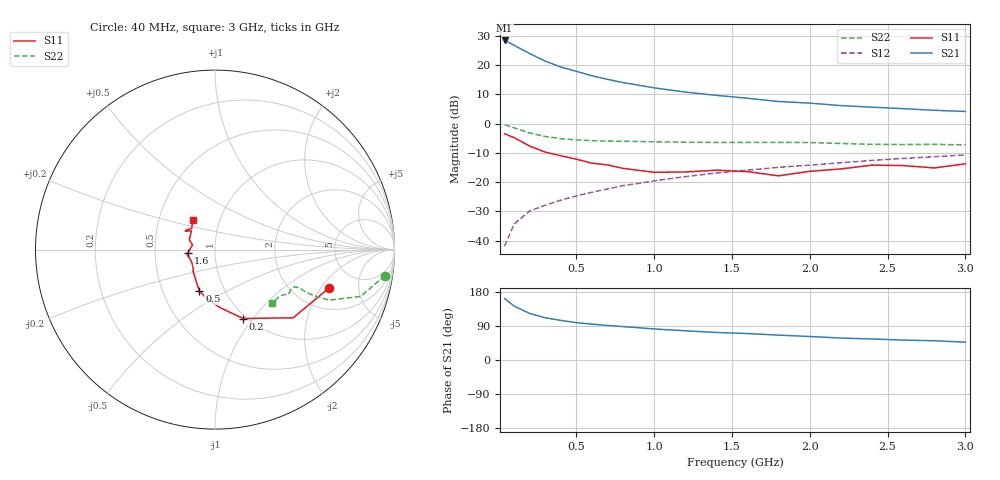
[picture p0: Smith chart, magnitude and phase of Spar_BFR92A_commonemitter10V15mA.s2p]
! Filename:  BFR92AI.S2P  Version:  2.0
! NXP part #: BFR92A  Date: May 1990
! Bias condition: Vce=10V, Ic=15mA
#  MHz  S  MA  R  50
! Freq  S11  S21  S12  S22  !GUM [dB]
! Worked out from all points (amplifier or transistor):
!   21 points, 40 MHz to 3 GHz, reference 50 ohm
!   highest |S21| = 28.5 dB at 40 MHz (marker M1)
!   |S21| within 3 dB of that: start of sweep to 148.3 MHz
!   unconditionally stable (mu >= 1): 897.4 MHz to 2.424 GHz; 2.693 GHz to 2.853 GHz
!   at 300 MHz: K = 0.77, MSG = 24.7 dB, |S12| = -28.0 dB
!   at 1 GHz: K = 1.01, MAG = 15.2 dB, |S12| = -19.6 dB
!   at 3 GHz: K = 0.98, MSG = 7.4 dB, |S12| = -10.7 dB
!   S11 on the Smith chart (normalised r, x): 40 MHz: 3.11, -2.41; 200 MHz: 0.97, -0.90; 500 MHz: 0.76, -0.37; 1.6 GHz: 0.74, -0.03; 3 GHz: 0.74, +0.25
40  0.672 -18.4  26.59 162.4  0.008 77.9  0.958 -8.7
100  0.578 -41.1  22.06 142.4  0.019 69.8  0.853 -17.8
200  0.415 -67.7  15.88 123.0  0.032 69.8  0.695 -23.9
300  0.326 -84.7  11.83 111.6  0.04 68.6  0.604 -25.0
400  0.283 -97.6  9.353 104.5  0.049 70.2  0.555 -25.1
500  0.247 -110.7  7.884 98.6  0.058 70.0  0.527 -24.5
600  0.211 -119.1  6.622 94.7  0.067 71.7  0.512 -24.5
700  0.197 -123.3  5.747 91.3  0.076 73.6  0.503 -24.7
800  0.172 -135.1  5.06 88.1  0.087 73.4  0.499 -24.6
900  0.159 -139.5  4.561 85.2  0.095 74.8  0.496 -25.0
1000  0.147 -152.9  4.106 82.0  0.105 74.6  0.489 -25.1
1200  0.149 -160.4  3.476 77.1  0.124 74.6  0.482 -26.1
1400  0.16 -172.5  3.055 72.7  0.143 74.2  0.477 -28.1
1600  0.151 -173.3  2.723 69.8  0.16 74.0  0.478 -29.1
1800  0.128 168.0  2.396 65.6  0.179 74.0  0.478 -30.8
2000  0.153 159.3  2.249 62.0  0.195 73.2  0.476 -32.0
2200  0.168 141.5  2.04 57.9  0.214 72.8  0.458 -33.1
2400  0.195 148.3  1.915 55.5  0.235 71.6  0.443 -36.5
2600  0.192 144.7  1.809 52.5  0.254 70.8  0.44 -39.8
2800  0.175 137.8  1.694 50.8  0.272 70.3  0.443 -42.3
3000  0.205 127.6  1.619 47.0  0.292 69.0  0.433 -43.2
